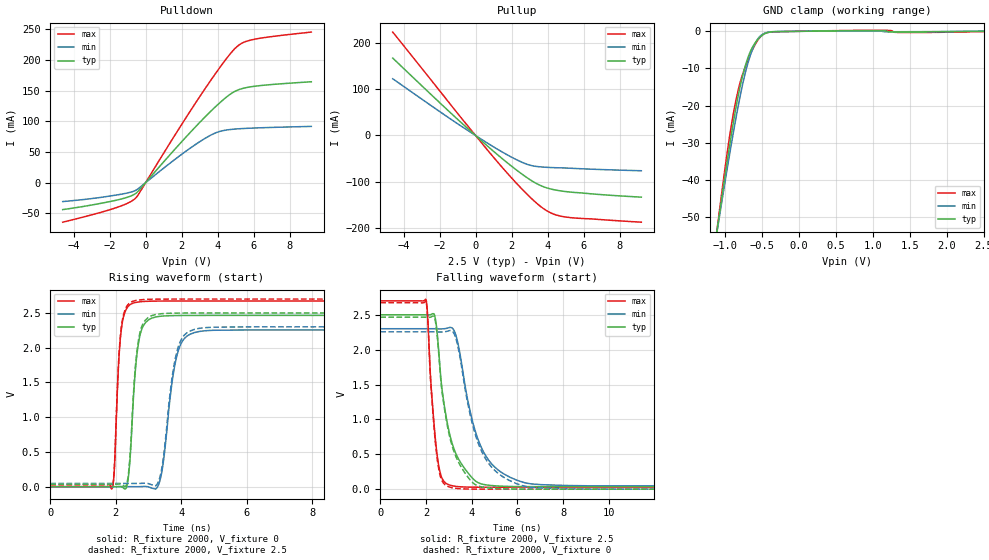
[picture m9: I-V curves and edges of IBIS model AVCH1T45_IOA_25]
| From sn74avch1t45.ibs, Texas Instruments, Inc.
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[Model]   AVCH1T45_IOA_25
Model_type  I/O
Vinl=0.7
Vinh=1.6
Enable   Active-Low
Vref =   0
Rref =   2000
Cref =   15p
Vmeas =   1.25
| variable   typ   min   max
C_comp   5.06pF   4.25pF   5.75pF
| C_pullup   4.25pF   3.21pF   5.63pF
| C_pulldown   4.37pF   3.82pF   4.80pF
| C_tri-state   5.06pF   4.25pF   5.75pF
[Temperature Range]   40   100   -40
| Ambient temperature   25   85   -40
[Voltage range]   2.5   2.3   2.7
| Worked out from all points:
|   slope of the pulldown table from 0 to 0.375 V, typ, clamps not added: 29.4 ohm
|   slope of the pullup table from 0 to 0.375 V, typ, clamps not added: 28.8 ohm
|   GND clamp passes 1 mA (typ) near -0.49 V on its own axis
|   rising waveform, R_fixture 2000, V_fixture 0: 20-80 % time 216ps typ, 348ps min, 158ps max; typ from 0 V to 2.46 V
|   falling waveform, R_fixture 2000, V_fixture 2.5: 20-80 % time 733ps typ, 1.05ns min, 342ps max; typ from 2.5 V to 0.036 V
|   rising waveform, R_fixture 2000, V_fixture 2.5: 20-80 % time 214ps typ, 345ps min, 157ps max; typ from 0.036 V to 2.5 V
|   falling waveform, R_fixture 2000, V_fixture 0: 20-80 % time 727ps typ, 1.05ns min, 334ps max; typ from 2.46 V to 0 V
[GND Clamp]
| AVCH1T45_IOA_25
|   Voltage   I(typ)   I(min)   I(max)
-4.6V     -599.7mA   -548.2mA   -664.8mA
-1.105V   -53.1mA    -53.46mA   -52.72mA
-1.08V    -49.64mA   -50.32mA   -48.82mA
-930mV    -29.72mA   -32.1mA    -27.1mA
-880mV    -23.65mA   -26.37mA   -21.29mA
-825mV    -17.62mA   -20.4mA    -16.07mA
-750mV    -11.02mA   -13.17mA   -10.85mA
-665mV    -5.769mA   -6.898mA   -6.554mA
-590mV    -3.043mA   -3.142mA   -3.475mA
-510mV    -1.266mA   -1.045mA   -1.273mA
-305mV    -86.62uA   -60.85uA   -133.1uA
2.5V      1.212nA    39.39uA    -82.83uA
[Pulldown]
| AVCH1T45_IOA_25
|   Voltage   I(typ)   I(min)   I(max)
-4.6V     -43.76mA   -30.71mA   -64.27mA
-1.715V   -29.08mA   -20.46mA   -41.45mA
-985mV    -23.44mA   -16.53mA   -33.24mA
-545mV    -17.41mA   -12.35mA   -24.86mA
1.85V     61.76mA    42.85mA    87.78mA
3.295V    106.9mA    72.08mA    152.8mA
4.12V     130.1mA    83.49mA    187.5mA
4.755V    145.2mA    86.77mA    211.8mA
5.15V     151.2mA    87.75mA    223.4mA
5.545V    154.6mA    88.42mA    229.7mA
6.15V     157.4mA    89.19mA    234.2mA
9.2V      164.4mA    91.67mA    245.2mA
[Pullup]
| AVCH1T45_IOA_25
|   Voltage   I(typ)   I(min)   I(max)
-4.6V     167.2mA    122.6mA    223.3mA
-1.155V   40.55mA    29.45mA    55.44mA
1.195V    -40.71mA   -29.18mA   -56.05mA
2.025V    -67.14mA   -47.36mA   -92.77mA
2.695V    -86.73mA   -59.71mA   -120.4mA
3.12V     -97.9mA    -65.07mA   -136.7mA
3.615V    -108.1mA   -67.81mA   -153.5mA
4.245V    -116.2mA   -69.29mA   -168.4mA
4.95V     -120.8mA   -70.1mA    -175.7mA
9.2V      -133.1mA   -76.13mA   -187.2mA
[Ramp]
| AVCH1T45_IOA_25
| variable   typ   min   max
dV/dt_r   1.50/2.21E-10   1.38/3.60E-10   1.62/1.63E-10
dV/dt_f   1.49/7.35E-10   1.36/1.05E-09   1.62/3.43E-10
R_load = 2000
[Rising Waveform]
| AVCH1T45_IOA_25
R_fixture =   2000
C_fixture =   0
L_fixture =   0
V_fixture =   0
V_fixture_min = 0
V_fixture_max = 0
|   Time   V(typ)   V(min)   V(max)
0s        27.66nV    106.2nV    1.086nV
1.895ns   31.36uV    -1.268uV   -19.06mV
2.175ns   42.58uV    -22.72uV   2.285V
2.385ns   138.5mV    35.54uV    2.598V
2.63ns    1.836V     -206.6uV   2.653V
2.835ns   2.31V      2.811mV    2.664V
3.31ns    2.449V     30.45mV    2.671V
3.875ns   2.463V     1.902V     2.672V
4.55ns    2.465V     2.234V     2.672V
29.99ns   2.465V     2.256V     2.672V
[Falling Waveform]
| AVCH1T45_IOA_25
R_fixture =   2000
C_fixture =   0
L_fixture =   0
V_fixture =   2.5
V_fixture_min = 2.3
V_fixture_max = 2.7
|   Time   V(typ)   V(min)   V(max)
0s        2.5V       2.3V       2.7V
1.995ns   2.499V     2.3V       2.722V
2.355ns   2.512V     2.3V       923.5mV
2.5ns     2.207V     2.298V     463.3mV
2.715ns   1.399V     2.298V     148.1mV
3.085ns   725.2mV    2.319V     54.31mV
3.355ns   477.2mV    2.152V     38.56mV
4.44ns    73.83mV    586mV      27.8mV
6.295ns   36.52mV    94.71mV    27.4mV
29.99ns   35.81mV    46.58mV    27.39mV
[Rising Waveform]
| AVCH1T45_IOA_25
R_fixture =   2000
C_fixture =   0
L_fixture =   0
V_fixture =   2.5
V_fixture_min = 2.3
V_fixture_max = 2.7
|   Time   V(typ)   V(min)   V(max)
0s        35.81mV    46.58mV    27.38mV
1.895ns   35.84mV    46.58mV    8.36mV
2.17ns    36.7mV     46.56mV    2.298V
2.385ns   175.8mV    46.62mV    2.627V
2.625ns   1.858V     46.37mV    2.681V
2.83ns    2.344V     49.31mV    2.692V
3.31ns    2.485V     78.67mV    2.699V
3.865ns   2.498V     1.943V     2.7V
4.535ns   2.5V       2.278V     2.7V
29.99ns   2.5V       2.3V       2.7V
[Falling Waveform]
| AVCH1T45_IOA_25
R_fixture =   2000
C_fixture =   0
L_fixture =   0
V_fixture =   0
V_fixture_min = 0
V_fixture_max = 0
|   Time   V(typ)   V(min)   V(max)
0s        2.465V     2.256V     2.672V
1.995ns   2.464V     2.256V     2.695V
2.355ns   2.477V     2.256V     879.5mV
2.495ns   2.189V     2.254V     425mV
2.71ns    1.381V     2.254V     115.7mV
3.08ns    695.8mV    2.275V     25.72mV
3.35ns    437.9mV    2.112V     10.53mV
4.435ns   32.19mV    542.8mV    385.6uV
6.26ns    606.4uV    47.03mV    15.11uV
29.99ns   422nV      402.9nV    244.4nV
